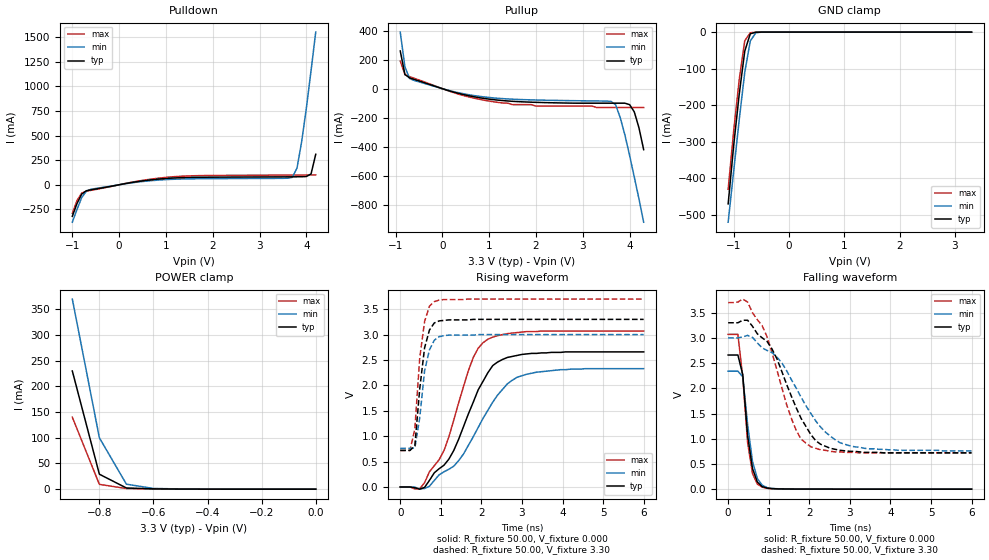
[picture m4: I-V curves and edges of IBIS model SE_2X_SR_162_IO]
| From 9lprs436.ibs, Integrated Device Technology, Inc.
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|   Model SE_2X_SR_162_IO
[Model]   SE_2X_SR_162_IO
Model_type   I/O
Polarity   Inverting
Vinl =   0.80V
Vinh =   2.00V
Vmeas =   1.50V
Cref =   5.00pF
Rref =  0.000
Vref =   1.50V
C_comp   3.40pF   2.85pF   3.95pF
[Temperature Range]   27.00   70.00   0.000
[Voltage Range]   3.30V   3.00V   3.70V
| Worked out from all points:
|   slope of the pulldown table from 0 to 0.495 V, typ, clamps not added: 12.7 ohm
|   slope of the pullup table from 0 to 0.495 V, typ, clamps not added: 11.3 ohm
|   GND clamp passes 1 mA (typ) near -0.61 V on its own axis
|   POWER clamp passes 1 mA (typ) near -0.62 V on its own axis
|   rising waveform, R_fixture 50.00, V_fixture 0.000: 20-80 % time 892ps typ, 1.08ns min, 747ps max; typ from 0 V to 2.66 V
|   rising waveform, R_fixture 50.00, V_fixture 3.30: 20-80 % time 209ps typ, 228ps min, 199ps max; typ from 0.72 V to 3.3 V
|   falling waveform, R_fixture 50.00, V_fixture 0.000: 20-80 % time 203ps typ, 224ps min, 214ps max; typ from 2.66 V to 0 V
|   falling waveform, R_fixture 50.00, V_fixture 3.30: 20-80 % time 846ps typ, 1.03ns min, 688ps max; typ from 3.3 V to 0.72 V
[Pulldown]
| voltage   I(typ)   I(min)   I(max)
|  -3.30   -4.16A   -4.01A   -4.26A
|  -3.10   -3.82A   -3.69A   -3.90A
|  -2.90   -3.48A   -3.37A   -3.55A
|  -2.70   -3.14A   -3.05A   -3.20A
|  -2.50   -2.80A   -2.72A   -2.85A
|  -2.30   -2.46A   -2.41A   -2.50A
|  -2.10   -2.12A   -2.09A   -2.15A
|  -1.90   -1.79A   -1.77A   -1.80A
|  -1.70   -1.45A   -1.45A   -1.45A
|  -1.50   -1.12A   -1.14A   -1.11A
-1V       -320mA     -380mA     -290mA
-900mV    -190mA     -250mA     -160mA
-800mV    -94.75mA   -130mA     -84.77mA
-700mV    -60.71mA   -64.75mA   -65.52mA
-600mV    -51.06mA   -45.2mA    -56.5mA
1.2V      69.5mA     56.57mA    82.87mA
3.7V      80.56mA    75.15mA    98.32mA
3.8V      80.96mA    170mA      98.58mA
3.9V      81.72mA    440mA      98.88mA
4V        83.73mA    780mA      99.22mA
4.1V      110mA      1.16A      99.62mA
4.2V      310mA      1.55A      100mA
|   4.30   0.66A   1.95A   0.10A
|   4.50   1.46A   2.77A   0.11A
|   4.70   2.32A   3.60A   0.58A
|   4.90   3.19A   4.43A   1.41A
|   5.10   4.07A   5.27A   2.30A
|   5.30   4.96A   6.12A   3.20A
|   5.50   5.85A   6.96A   4.12A
|   5.70   6.75A   7.81A   5.04A
|   5.90   7.65A   8.66A   5.97A
|   6.10   8.55A   9.52A   6.90A
|   6.60   10.81A   11.65A   9.23A
[Pullup]
| voltage   I(typ)   I(min)   I(max)
|  -3.30   10.68A   10.27A   10.94A
|  -3.10   9.79A   9.43A   10.01A
|  -2.90   8.89A   8.58A   9.09A
|  -2.70   7.99A   7.73A   8.16A
|  -2.50   7.10A   6.88A   7.23A
|  -2.30   6.20A   6.04A   6.31A
|  -2.10   5.31A   5.20A   5.38A
|  -1.90   4.43A   4.36A   4.47A
|  -1.70   3.54A   3.53A   3.55A
|  -1.50   2.67A   2.70A   2.64A
|  -1.00   0.59A   0.73A   0.50A
-900mV    260mA      390mA      190mA
-800mV    98.15mA    150mA      96.76mA
-700mV    74.35mA    69.94mA    82.79mA
-600mV    63.81mA    56.49mA    71.52mA
500mV     -44.25mA   -37.82mA   -51.47mA
1.5V      -86.95mA   -72.42mA   -110mA
3.5V      -100mA     -85.41mA   -130mA
3.7V      -100mA     -110mA     -130mA
3.9V      -100mA     -320mA     -130mA
4.1V      -160mA     -610mA     -130mA
4.2V      -270mA     -760mA     -130mA
4.3V      -420mA     -920mA     -130mA
|   4.50   -0.73A   -1.22A   -0.15A
|   4.70   -1.06A   -1.54A   -0.40A
|   4.90   -1.39A   -1.86A   -0.73A
|   5.10   -1.72A   -2.17A   -1.06A
|   5.30   -2.06A   -2.49A   -1.41A
|   5.50   -2.40A   -2.81A   -1.75A
|   5.70   -2.74A   -3.13A   -2.10A
|   5.90   -3.07A   -3.46A   -2.45A
|   6.10   -3.41A   -3.78A   -2.80A
|   6.60   -4.27A   -4.58A   -3.68A
[GND_clamp]
| voltage   I(typ)   I(min)   I(max)
|  -3.30   -4.16A   -4.01A   -4.26A
|  -3.20   -3.99A   -3.85A   -4.08A
|  -3.10   -3.82A   -3.69A   -3.90A
|  -3.00   -3.65A   -3.53A   -3.73A
|  -2.90   -3.48A   -3.37A   -3.55A
|  -2.80   -3.31A   -3.20A   -3.37A
|  -2.70   -3.14A   -3.04A   -3.20A
|  -2.60   -2.97A   -2.88A   -3.02A
|  -2.50   -2.80A   -2.72A   -2.85A
|  -2.40   -2.63A   -2.56A   -2.67A
|  -2.30   -2.46A   -2.40A   -2.49A
|  -2.20   -2.29A   -2.24A   -2.32A
|  -2.10   -2.12A   -2.09A   -2.14A
|  -2.00   -1.95A   -1.93A   -1.97A
|  -1.90   -1.78A   -1.77A   -1.80A
|  -1.80   -1.62A   -1.61A   -1.62A
|  -1.70   -1.45A   -1.45A   -1.45A
|  -1.60   -1.28A   -1.29A   -1.27A
|  -1.50   -1.12A   -1.14A   -1.10A
|  -1.40   -0.95A   -0.98A   -0.93A
|  -1.30   -0.79A   -0.83A   -0.76A
|  -1.20   -0.63A   -0.67A   -0.59A
-1.1V     -470mA     -520mA     -430mA
-1V       -310mA     -380mA     -270mA
-900mV    -170mA     -240mA     -130mA
-800mV    -52.15mA   -110mA     -23.62mA
-700mV    -4.69mA    -24.32mA   -1.84mA
-600mV    -430uA     -1.9mA     -210uA
-400mV    -1.76uA    -10.15uA   -470nA
3.3V      150pA      19.33uA    -230pA
[POWER_clamp]
| voltage   I(typ)   I(min)   I(max)
|  -3.30   10.68A   10.27A   10.94A
|  -3.20   10.23A   9.85A   10.48A
|  -3.10   9.78A   9.43A   10.01A
|  -3.00   9.34A   9.00A   9.55A
|  -2.90   8.89A   8.58A   9.09A
|  -2.80   8.44A   8.15A   8.62A
|  -2.70   7.99A   7.73A   8.16A
|  -2.60   7.54A   7.31A   7.69A
|  -2.50   7.10A   6.88A   7.23A
|  -2.40   6.65A   6.46A   6.77A
|  -2.30   6.20A   6.04A   6.31A
|  -2.20   5.76A   5.62A   5.84A
|  -2.10   5.31A   5.20A   5.38A
|  -2.00   4.87A   4.78A   4.92A
|  -1.90   4.42A   4.36A   4.46A
|  -1.80   3.98A   3.94A   4.00A
|  -1.70   3.54A   3.53A   3.55A
|  -1.60   3.10A   3.11A   3.09A
|  -1.50   2.67A   2.70A   2.64A
|  -1.40   2.23A   2.29A   2.19A
|  -1.30   1.80A   1.88A   1.75A
|  -1.20   1.38A   1.48A   1.31A
|  -1.10   0.97A   1.09A   0.88A
|  -1.00   0.57A   0.72A   0.48A
-900mV    230mA      370mA      140mA
-800mV    29.1mA     100mA      9.35mA
-700mV    2.27mA     9.67mA     1.22mA
-600mV    610uA      1.4mA      350uA
-500mV    160uA      410uA      72.16uA
-400mV    29.46uA    100uA      11.5uA
-300mV    4.41uA     19.33uA    1.4uA
-200mV    480nA      2.95uA     110nA
-100mV    32.67nA    310nA      5.63nA
0V        150pA      200pA      170pA
[Ramp]
| variable   typ   min   max
dV/dt_r   1.60/0.89n   1.40/1.08n   1.84/0.74n
dV/dt_f   1.55/0.84n   1.34/1.03n   1.79/0.68n
R_load = 50.00
[Rising Waveform]
R_fixture = 50.00
V_fixture = 0.000
V_fixture_min = 0.000
V_fixture_max = 0.000
| time   V(typ)   V(min)   V(max)
0s        0V         1.34uV     0V
480ps     -43.18mV   -35.91mV   -37.17mV
720ps     130mV      14.25mV    300mV
960ps     360mV      240mV      540mV
1.32ns    720mV      410mV      1.32V
1.8ns     1.67V      990mV      2.55V
2.16ns    2.25V      1.51V      2.91V
2.64ns    2.55V      2.03V      3.02V
3.12ns    2.62V      2.22V      3.06V
6ns       2.66V      2.33V      3.07V
[Rising Waveform]
R_fixture = 50.00
V_fixture = 3.30
V_fixture_min = 3.00
V_fixture_max = 3.70
| time   V(typ)   V(min)   V(max)
0s        720mV      760mV      720mV
240ps     720mV      760mV      720mV
360ps     810mV      770mV      1.14V
480ps     1.93V      1.36V      2.54V
600ps     2.74V      2.29V      3.26V
720ps     3.09V      2.7V       3.56V
840ps     3.23V      2.89V      3.65V
960ps     3.27V      2.96V      3.68V
1.2ns     3.29V      2.99V      3.69V
6ns       3.3V       3V         3.7V
[Falling Waveform]
R_fixture = 50.00
V_fixture = 0.000
V_fixture_min = 0.000
V_fixture_max = 0.000
| time   V(typ)   V(min)   V(max)
0s        2.66V      2.34V      3.07V
240ps     2.66V      2.34V      3.07V
360ps     2.27V      2.23V      2.22V
480ps     1.06V      1.28V      920mV
600ps     410mV      550mV      310mV
720ps     140mV      210mV      100mV
840ps     50.65mV    77.82mV    38.04mV
960ps     22.32mV    31.12mV    16.68mV
1.32ns    4.45mV     6.2mV      3.18mV
6ns       1.35uV     5.89uV     0V
[Falling Waveform]
R_fixture = 50.00
V_fixture = 3.30
V_fixture_min = 3.00
V_fixture_max = 3.70
| time   V(typ)   V(min)   V(max)
0s        3.3V       3V         3.7V
480ps     3.35V      3.05V      3.71V
840ps     3V         2.8V       3.24V
1.2ns     2.59V      2.62V      2.37V
1.44ns    2.08V      2.35V      1.68V
1.68ns    1.61V      2V         1.16V
2.04ns    1.08V      1.5V       840mV
2.4ns     850mV      1.13V      770mV
3ns       750mV      860mV      730mV
6ns       720mV      760mV      720mV
